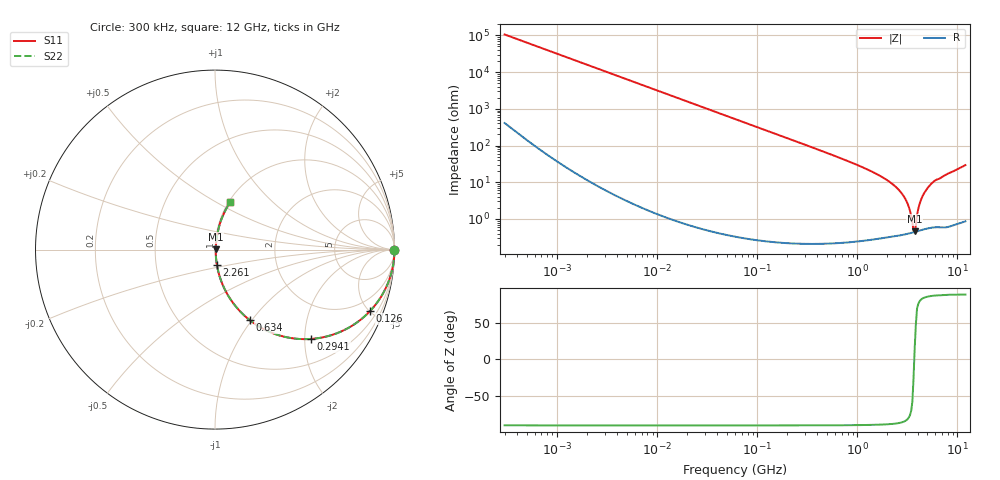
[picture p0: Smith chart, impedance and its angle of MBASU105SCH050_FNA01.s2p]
! MBASU105SCH050_FNA01  S-PARAMETER MODEL  ( Standard Model )
! Model Generated by TAIYO YUDEN Corporation (http://www.ty-top.com)
! Version 1.0
! TAIYO YUDEN Control No. 230609
! Copyright(c) 2023 TAIYO YUDEN CO.,LTD. All Rights Reserved.
! Product Description (link to TY-COMPAS)
! https://ds.yuden.co.jp/TYCOMPAS/or/detail?pn=MBASU105SCH050BFNA01&u=M
! Products Name : Multilayer Ceramic Capacitors
! Characteristics :
!  Capacitance : 5 [pF] , Rated Voltage : 50 [V] , TCC : CH / C0H
!  Case Size : 1.0 x 0.5 / 0.039 x 0.02 [mm/inch] , Thickness : 0.5 / 0.02 [mm/inch]
!  (Conditions: Temperature = 25 [degC] , DC Bias Voltage = 0 [V])
! External Node Assignments :
!  1  o---| |---o  2
! GND o---------o GND
! Frequency Range : 0.3MHz  -  12000MHz  [ 401 STEP ]
# MHZ S RI R 50
! Freq[MHz].  S11 Real  S11 Imag  S21 Real  S21 Imag  S12 Real  S12 Imag  S22 Real  S22 Imag
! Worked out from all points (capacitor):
!   401 points, 300 kHz to 12 GHz, reference 50 ohm
!   read as one part in series: C = 5 pF near 316.3 kHz
!   lowest |Z| = 458 mohm at 3.741 GHz (marker M1)
!   series resonance near 3.704 GHz, so ESL is about 370 pH
!   S11 on the Smith chart (normalised r, x): 300 kHz: open; 126 MHz: 1.00, -5.05; 294.1 MHz: 1.00, -2.15; 634 MHz: 1.00, -0.97; 2.261 GHz: 1.01, -0.18; 12 GHz: 1.02, +0.59
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0.3  1 -0.000942  4.54e-06 0.000942  4.54e-06 0.000942  1 -0.000942
1.769972  1 -0.00556  3.52e-05 0.00556  3.52e-05 0.00556  1 -0.00556
10.44266  0.9989 -0.0328  0.00109 0.0328  0.00109 0.0328  0.9989 -0.0328
60  0.9656 -0.182  0.0344 0.182  0.0344 0.182  0.9656 -0.182
125.9782  0.8641 -0.3422  0.1359 0.3422  0.1359 0.3422  0.8641 -0.3422
294.0765  0.5363 -0.4977  0.4637 0.4977  0.4637 0.4977  0.5363 -0.4977
353.9943  0.4426 -0.4955  0.5574 0.4955  0.5574 0.4955  0.4426 -0.4955
634.0297  0.1929 -0.3923  0.8071 0.3923  0.8071 0.3923  0.1929 -0.3923
1262.535  0.0494 -0.211  0.9506 0.211  0.9506 0.211  0.0494 -0.211
2088.533  0.0137 -0.1017  0.9863 0.1017  0.9863 0.1017  0.0137 -0.1017
2261.293  0.0109 -0.0865  0.9891 0.0865  0.9891 0.0865  0.0109 -0.0865
2650.866  0.00686 -0.0574  0.9931 0.0574  0.9931 0.0574  0.00686 -0.0574
3026.31  0.00497 -0.034  0.995 0.034  0.995 0.034  0.00497 -0.034
3276.641  0.00441 -0.0202  0.9956 0.0202  0.9956 0.0202  0.00441 -0.0202
3547.679  0.00427 -0.00653  0.9957 0.00653  0.9957 0.00653  0.00427 -0.00653
3740.715  0.00439 0.0012  0.9956 -0.0012  0.9956 -0.0012  0.00439 0.0012
3841.137  0.00451 0.00489  0.9955 -0.00489  0.9955 -0.00489  0.00451 0.00489
4158.869  0.00534 0.0236  0.9947 -0.0236  0.9947 -0.0236  0.00534 0.0236
4385.161  0.00628 0.0358  0.9937 -0.0358  0.9937 -0.0358  0.00628 0.0358
5278.635  0.0121 0.0799  0.9879 -0.0799  0.9879 -0.0799  0.0121 0.0799
6026.253  0.0184 0.1108  0.9816 -0.1108  0.9816 -0.1108  0.0184 0.1108
12000  0.0859 0.2659  0.9141 -0.2659  0.9141 -0.2659  0.0859 0.2659
